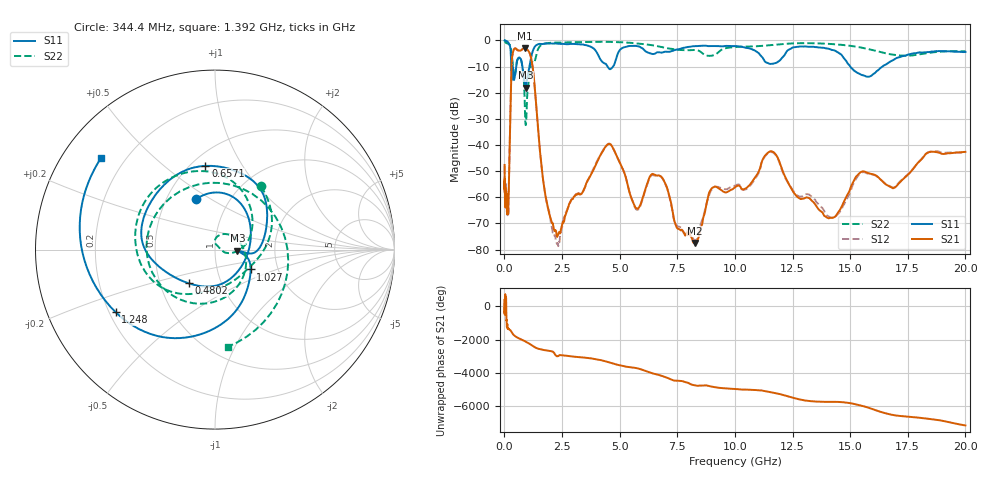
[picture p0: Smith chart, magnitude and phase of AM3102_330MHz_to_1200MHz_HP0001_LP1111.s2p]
! Date/Time: Tue, Sep 11, 2018 5:10 PM
! Network Analyzer: Agilent Technologies E8362B Rev: A.07.50.63
! Sweep from 0.010 to 20.000 GHz, 1601 Points, Sweep Type: LOG
! Power Supply: 4.949 V, 0.001 A
# Hz S DB R 50
!freq MagS11 AngS11 MagS21 AngS21 MagS12 AngS12 MagS22 AngS22
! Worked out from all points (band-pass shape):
!   1601 points, 10 MHz to 20 GHz, reference 50 ohm
!   highest |S21| = -2.97 dB at 886.4 MHz (marker M1); lowest = -77.5 dB at 8.266 GHz (marker M2)
!   |S21| within 3 dB of the highest: 341.3 MHz to 1.138 GHz (796.5 MHz wide, 108 % of centre)
!   lowest |S11| = -18.0 dB at 920.7 MHz (marker M3), VSWR 1.29, Z = 64.3 - j0.718 ohm
!   |S11| at or under -10 dB: 781.1 MHz to 1.086 GHz (304.9 MHz wide, 32.7 % of centre); 4.475 GHz to 4.713 GHz (237.4 MHz wide, 5.17 % of centre); 15.01 GHz to 16.4 GHz (1.392 GHz wide, 8.87 % of centre)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
!   |S22| runs from -32.4 to -0.3 dB; largest |S21 - S12| = 0.012
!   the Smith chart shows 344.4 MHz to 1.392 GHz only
!   S11 on the Smith chart (normalised r, x): 344.4 MHz: 0.70, +0.43; 480.2 MHz: 0.70, -0.28; 657.1 MHz: 0.59, +0.70; 1.027 GHz: 1.45, -0.34; 1.248 GHz: 0.23, -0.27; 1.392 GHz: 0.11, +0.35
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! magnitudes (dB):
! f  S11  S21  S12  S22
! 10 MHz  0.0  -47.6  -48.1  -0.3
! 35.55 MHz  0.0  -63.6  -61.8  -0.6
! 126.4 MHz  -0.4  -66.1  -64.0  -1.1
! 175.4 MHz  -0.9  -62.7  -64.0  -1.3
! 344.4 MHz  -10.4  -5.8  -5.9  -7.2
! 447.2 MHz  -14.1  -3.1  -3.1  -13.7
! 480.2 MHz  -12.5  -3.0  -3.1  -12.2
! 657.1 MHz  -6.6  -3.9  -4.0  -6.5
! 886.4 MHz  -16.7  -3.0  -3.0  -25.0
! 920.7 MHz  -18.0  -3.0  -3.1  -32.2
! 1.027 GHz  -12.9  -3.8  -3.8  -17.6
! 1.248 GHz  -3.7  -11.6  -11.7  -8.5
! 1.392 GHz  -1.8  -26.0  -26.4  -5.3
! 1.59 GHz  -1.4  -46.3  -46.2  -1.8
! 2.303 GHz  -1.2  -74.9  -77.5  -0.8
! 4.479 GHz  -10.0  -39.9  -39.7  -0.5
! 5.652 GHz  -2.1  -63.4  -63.7  -1.0
! 6.643 GHz  -4.5  -51.7  -51.6  -2.2
! 8.266 GHz  -2.2  -77.5  -76.5  -3.6
! 11.47 GHz  -8.8  -42.7  -42.9  -1.9
! 14.07 GHz  -3.2  -68.0  -67.3  -1.3
! 20 GHz  -4.4  -42.6  -43.1  -4.1
